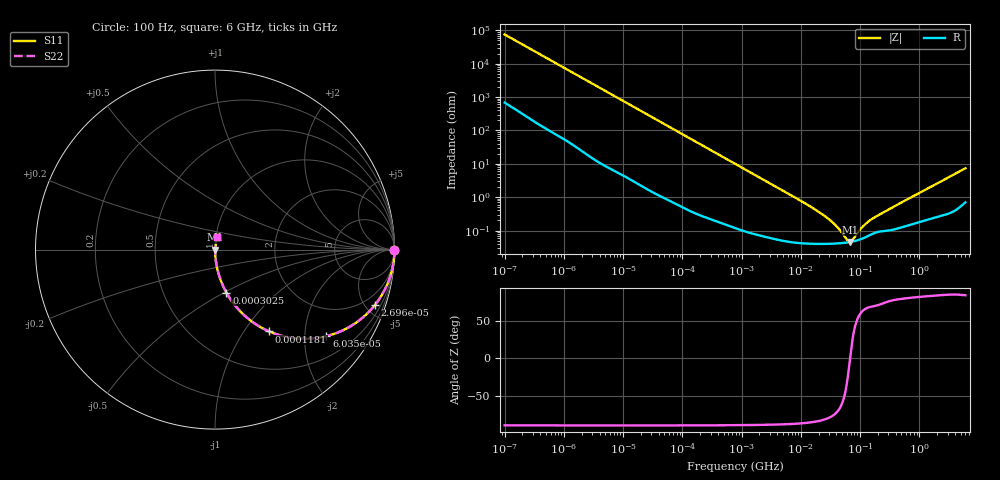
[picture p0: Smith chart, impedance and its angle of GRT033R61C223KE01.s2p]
!Murata Part Number: GRT033R61C223KE01
!These Parameters are Measured in Series Mode Connection
!Data Generated on Jun 19, 2026
!  o--ll--o
!Port1  Port2
!  o------o
!Operation Temp=25[degC], DC Bias Voltage=0[V]
!Freq. Start=100[Hz] Stop=6[GHz] 401[Steps]
# Hz S RI R 50
!Freq.(Hz) S11(Real) S11(Imag) S21(Real) S21(Imag) S12(Real) S12(Imag) S22(Real) S22(Imag)
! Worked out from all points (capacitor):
!   401 points, 100 Hz to 6 GHz, reference 50 ohm
!   read as one part in series: C = 21.1 nF near 109 Hz
!   lowest |Z| = 45.3 mohm at 68.17 MHz (marker M1)
!   series resonance near 67.81 MHz, so ESL is about 260 pH
!   S11 on the Smith chart (normalised r, x): 100 Hz: open; 26.96 kHz: 1.03, -5.72; 60.35 kHz: 1.02, -2.56; 118.1 kHz: 1.01, -1.31; 302.5 kHz: 1.00, -0.51; 6 GHz: 1.01, +0.15
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100  1 -0.00133  1.38e-05 0.00133  1.38e-05 0.00133  1 -0.00133
2008  0.9991 -0.0263  0.000857 0.0263  0.000857 0.0263  0.9991 -0.0263
8801  0.9864 -0.113  0.0136 0.113  0.0136 0.113  0.9864 -0.113
26957  0.8896 -0.3105  0.1104 0.3105  0.1104 0.3105  0.8896 -0.3105
40335  0.7841 -0.4085  0.2159 0.4085  0.2159 0.4085  0.7841 -0.4085
60352  0.6206 -0.4822  0.3794 0.4822  0.3794 0.4822  0.6206 -0.4822
82567  0.4679 -0.4958  0.5321 0.4958  0.5321 0.4958  0.4679 -0.4958
118133  0.302 -0.4559  0.698 0.4559  0.698 0.4559  0.302 -0.4559
184852  0.1516 -0.3551  0.8484 0.3551  0.8484 0.3551  0.1516 -0.3551
302498  0.0637 -0.2401  0.9363 0.2401  0.9363 0.2401  0.0637 -0.2401
774597  0.0112 -0.0996  0.9888 0.0996  0.9888 0.0996  0.0112 -0.0996
2481164  0.00165 -0.0316  0.9984 0.0316  0.9984 0.0316  0.00165 -0.0316
1.555665e7  0.000423 -0.00482  0.9996 0.00482  0.9996 0.00482  0.000423 -0.00482
3.330331e7  0.000405 -0.0018  0.9996 0.0018  0.9996 0.0018  0.000405 -0.0018
4.35672e7  0.000413 -0.00106  0.9996 0.00106  0.9996 0.00106  0.000413 -0.00106
5.960426e7  0.000436 -0.0003  0.9996 0.0003  0.9996 0.0003  0.000436 -0.0003
6.817316e7  0.000453 1.27e-05  0.9995 -1.27e-05  0.9995 -1.27e-05  0.000453 1.27e-05
7.455971e7  0.000467 0.00022  0.9995 -0.00022  0.9995 -0.00022  0.000467 0.00022
1.020051e8  0.000547 0.000962  0.9995 -0.000962  0.9995 -0.000962  0.000547 0.000962
1.334425e8  0.000672 0.00163  0.9993 -0.00163  0.9993 -0.00163  0.000672 0.00163
3.124326e8  0.00102 0.00425  0.999 -0.00425  0.999 -0.00425  0.00102 0.00425
6e9  0.0121 0.0715  0.9879 -0.0715  0.9879 -0.0715  0.0121 0.0715
